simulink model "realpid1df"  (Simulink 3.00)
settings: Solver=ode45  SolverMode=SingleTasking  StartTime=0.0  StopTime=50  FixedStep=st_size  MaxStep=st_size  RelTol=1e-5  AbsTol=1e-6
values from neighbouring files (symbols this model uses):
  d_through_p = get(MAIN_MENU(19),'Value')    [cback.m]    (also in imcmenu.m = 0)
  Disturb = Setpoint    [mimo_MSF1DF_sim.m]    (also in mimo_MSF2DF_sim.m)
  K = 1/kpd    [imc2pseucon.m]    (also in imc2pseudo.m)
  Satlb = temp1    [cback.m]    (also in imcmenu.m = str2num(satlbs))
  Satub = temp1    [cback.m]    (also in imcmenu.m = str2num(satubs))
  Setpoint = zeros(1,n)    [mimo_MSF1DF_sim.m]    (also in mimo_MSF2DF_sim.m)
undefined symbols (not defined in the file or in its folder): denPd, denPs, numPd, numPs, TauD, TauI
libraries: MIMO_lib x1

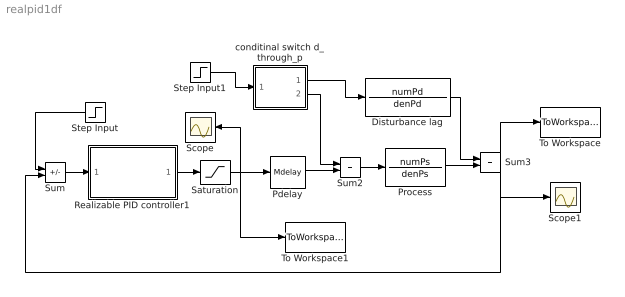
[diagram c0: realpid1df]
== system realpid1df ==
  Disturbance lag : TransferFcn  Numerator=numPd  Denominator=denPd
  Pdelay : MIMO_lib/Mdelay  Mdelay=Pdelay
  Process : TransferFcn  Numerator=numPs  Denominator=denPs
  Realizable PID controller1 : Subsystem
  Saturation : Saturate  UpperLimit=Satub  LowerLimit=Satlb
  Scope : Scope
  Scope1 : Scope
  Step Input : Step  Orientation=left  Time=0  Before=0  After=Setpoint  SampleTime=0
  Step Input1 : Step  Time=0  Before=0  After=Disturb  SampleTime=0
  Sum : Sum  Inputs=+-  SaturateOnIntegerOverflow=on
  Sum2 : Sum  Inputs=++  SaturateOnIntegerOverflow=on
  Sum3 : Sum  Inputs=++  SaturateOnIntegerOverflow=on
  To Workspace : ToWorkspace  VariableName=simout  SampleTime=-1  SaveFormat=Matrix
  To Workspace1 : ToWorkspace  VariableName=effort  SampleTime=-1  SaveFormat=Matrix
  conditinal switch d_through_p : Subsystem  Description=pass input signal through out1 if condition is true.
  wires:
  Sum/1 -> Realizable PID controller1/1(In1)
  Step Input/1 -> Sum/1
  Realizable PID controller1/1(Out1) -> Saturation/1
  Saturation/1 -> Pdelay/1, Scope/1, To Workspace1/1
  conditinal switch d_through_p/1(Out2) -> Disturbance lag/1
  conditinal switch d_through_p/2(Out1) -> Sum2/1
  Step Input1/1 -> conditinal switch d_through_p/1(In)
  Pdelay/1 -> Sum2/2
  Sum2/1 -> Process/1
  Process/1 -> Sum3/2
  Disturbance lag/1 -> Sum3/1
  Sum3/1 -> Sum/2, To Workspace/1, Scope1/1

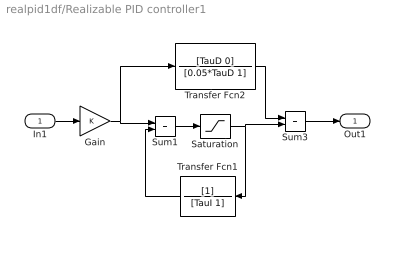
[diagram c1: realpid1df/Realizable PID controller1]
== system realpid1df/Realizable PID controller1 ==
  In1 : Inport  Port=1  PortWidth=-1  SampleTime=-1  DataType=auto
  Gain : Gain  Gain=K  SaturateOnIntegerOverflow=on
  Saturation : Saturate  UpperLimit=Satub  LowerLimit=Satlb
  Sum1 : Sum  Inputs=++  SaturateOnIntegerOverflow=on
  Sum3 : Sum  Inputs=++  SaturateOnIntegerOverflow=on
  Transfer Fcn1 : TransferFcn  Orientation=left  Numerator=[1]  Denominator=[TauI 1]
  Transfer Fcn2 : TransferFcn  Numerator=[TauD 0]  Denominator=[0.05*TauD 1]
  Out1 : Outport  Port=1  InitialOutput=0
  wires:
  Sum1/1 -> Saturation/1
  Transfer Fcn1/1 -> Sum1/2
  Gain/1 -> Sum1/1, Transfer Fcn2/1
  Transfer Fcn2/1 -> Sum3/1
  Sum3/1 -> Out1/1
  In1/1 -> Gain/1
  Saturation/1 -> Sum3/2, Transfer Fcn1/1

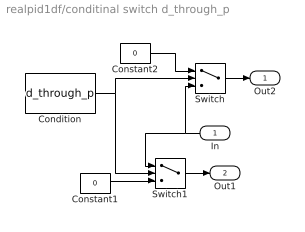
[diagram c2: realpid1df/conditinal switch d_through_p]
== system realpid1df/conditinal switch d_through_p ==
  In : Inport  Orientation=left  Port=1  PortWidth=-1  SampleTime=-1  DataType=auto
  Condition : Constant  Value=d_through_p
  Constant1 : Constant  Value=0
  Constant2 : Constant  Value=0
  Switch : Switch  Threshold=1
  Switch1 : Switch  Threshold=1
  Out2 : Outport  Port=1  InitialOutput=0
  Out1 : Outport  Port=2  InitialOutput=0
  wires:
  In/1 -> Switch/3, Switch1/1
  Condition/1 -> Switch1/2, Switch/2
  Constant1/1 -> Switch1/3
  Constant2/1 -> Switch/1
  Switch/1 -> Out2/1
  Switch1/1 -> Out1/1
